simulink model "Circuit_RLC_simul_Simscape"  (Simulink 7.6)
settings: Solver=ode15s  StartTime=0.0  StopTime=0.14  RelTol=1e-3
InitFcn:
  | % paramètres du circuit RLC
  | R=1;
  | L=0.01;
  | C=1e-3;
  | 
  | % fonction de transfert du 2nd ordre
  | dzeta=R*sqrt(C/L)/2;
  | w0=1/sqrt(L*C);
StopFcn:
  | close all, clc
  | load  VC_circuit_RLC_Simscape.mat
  | plot(x(1,:),x(2,:))
  | hold on
  | plot(x(1,:),x(3,:))
  | axis([0 0.14 -0.2 1.7])
  | grid
  | title('Tension aux bornes de C et échelon d''entrée')
  | xlabel('Circuit RLC - Simulation de l''inductance et de la capacité')
libraries: fl_lib x26, nesl_utility x5

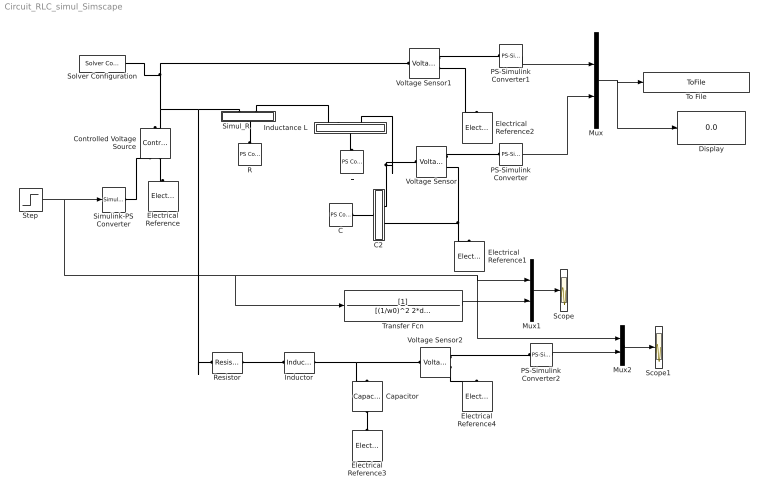
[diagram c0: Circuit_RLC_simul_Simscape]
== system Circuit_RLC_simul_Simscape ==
  C : fl_lib/Physical Signals/Sources/PS Constant  DialogController=NetworkEngine.DynNeDlgSource  SystemSampleTime=-1  constant=C  LocalVarLogging=[]
  C2 : Subsystem
  Capacitor : fl_lib/Electrical/Electrical Elements/Capacitor  DialogController=NetworkEngine.DynNeDlgSource  SystemSampleTime=-1  c=C F  v0=0 V  r=1e-6 Ohm  g=0 1/Ohm  i_Log=off  v_Log=off  vc_Log=off  LocalVarNames=|i|v|vc  LocalVarDescs=|i|v|Internal variable for voltage across capacitor term  LocalVarLogging=[0 0 0]
  Controlled Voltage Source : fl_lib/Electrical/Electrical Sources/Controlled Voltage Source  DialogController=NetworkEngine.DynNeDlgSource  SystemSampleTime=-1  i_Log=off  v_Log=off  LocalVarNames=|i|v  LocalVarDescs=|i|v  LocalVarLogging=[0 0]
  Display : Display
  Electrical Reference{,1..4} (5 alike) : fl_lib/Electrical/Electrical Elements/Electrical Reference  DialogController=NetworkEngine.DynNeDlgSource  SystemSampleTime=-1  i_Log=off  LocalVarNames=|i  LocalVarDescs=|i  LocalVarLogging=0
  "Inductance L  " : Subsystem  mask{L=0}
      mask prompts: L "Inductance"
  Inductor : fl_lib/Electrical/Electrical Elements/Inductor  DialogController=NetworkEngine.DynNeDlgSource  SystemSampleTime=-1  l=L H  i0=0 A  r=0 Ohm  g=1e-9 1/Ohm  i_Log=off  v_Log=off  i_L_Log=off  LocalVarNames=|i|v|i_L  LocalVarDescs=|i|v|Internal variable for current through inductor term  LocalVarLogging=[0 0 0]
  L : fl_lib/Physical Signals/Sources/PS Constant  DialogController=NetworkEngine.DynNeDlgSource  SystemSampleTime=-1  constant=L  LocalVarLogging=[]
  Mux : Mux  Inputs=2
  Mux1 : Mux  Inputs=2
  Mux2 : Mux  Inputs=2
  PS-Simulink Converter : nesl_utility/PS-Simulink Converter  DialogController=NetworkEngine.DynNeUtilDlgSource  SystemSampleTime=-1  PhysicalDomain=network_engine_domain  LeftPortType=input  RightPortType=output  SubClassName=ps_output  Unit=1  AffineConversion=off
  PS-Simulink Converter1 : nesl_utility/PS-Simulink Converter  DialogController=NetworkEngine.DynNeUtilDlgSource  SystemSampleTime=-1  PhysicalDomain=network_engine_domain  LeftPortType=input  RightPortType=output  SubClassName=ps_output  Unit=1  AffineConversion=off
  PS-Simulink Converter2 : nesl_utility/PS-Simulink Converter  DialogController=NetworkEngine.DynNeUtilDlgSource  SystemSampleTime=-1  PhysicalDomain=network_engine_domain  LeftPortType=input  RightPortType=output  SubClassName=ps_output  Unit=1  AffineConversion=off
  R : fl_lib/Physical Signals/Sources/PS Constant  DialogController=NetworkEngine.DynNeDlgSource  SystemSampleTime=-1  constant=R  LocalVarLogging=[]
  Resistor : fl_lib/Electrical/Electrical Elements/Resistor  DialogController=NetworkEngine.DynNeDlgSource  SystemSampleTime=-1  R=R Ohm  i_Log=off  v_Log=off  LocalVarNames=|i|v  LocalVarDescs=|i|v  LocalVarLogging=[0 0]
  Scope : Scope
  Scope1 : Scope
  Simul_R : Subsystem
  Simulink-PS Converter : nesl_utility/Simulink-PS Converter  DialogController=NetworkEngine.DynNeUtilDlgSource  SystemSampleTime=-1  PhysicalDomain=network_engine_domain  LeftPortType=input  RightPortType=output  SubClassName=ps_input  Unit=1  AffineConversion=off  InputFilterTimeConstant=.001  UdotUserProvided=0
  Solver Configuration : nesl_utility/Solver Configuration  DialogController=NetworkEngine.DynNeUtilDlgSource  SystemSampleTime=-1  PhysicalDomain=network_engine_domain  LeftPortType=input  RightPortType=generic  SubClassName=solver  Accelerate=off  Profile=off  ResidualTolerance=1e-9  MaxNonlinIter=3  MaxModeIter=2  DoFixedCost=off  UseLocalSampling=off  DoDC=off  LinearAlgebra=Sparse  LocalSolverSampleTime=.001  LocalSolverChoice=NE_BACKWARD_EULER_ADVANCER  UseLocalSolver=off
  Step : Step  Time=0.02  SampleTime=0
  To File : ToFile  Filename=VC_circuit_RLC_Simscape  MatrixName=x
  Transfer Fcn : TransferFcn  Denominator=[(1/w0)^2 2*dzeta/w0 1]
  Voltage Sensor : fl_lib/Electrical/Electrical Sensors/Voltage Sensor  DialogController=NetworkEngine.DynNeDlgSource  SystemSampleTime=-1  i1_Log=off  v1_Log=off  LocalVarNames=|i1|v1  LocalVarDescs=|i1|v1  LocalVarLogging=[0 0]
  Voltage Sensor1 : fl_lib/Electrical/Electrical Sensors/Voltage Sensor  DialogController=NetworkEngine.DynNeDlgSource  SystemSampleTime=-1  i1_Log=off  v1_Log=off  LocalVarNames=|i1|v1  LocalVarDescs=|i1|v1  LocalVarLogging=[0 0]
  Voltage Sensor2 : fl_lib/Electrical/Electrical Sensors/Voltage Sensor  DialogController=NetworkEngine.DynNeDlgSource  SystemSampleTime=-1  i1_Log=off  v1_Log=off  LocalVarNames=|i1|v1  LocalVarDescs=|i1|v1  LocalVarLogging=[0 0]
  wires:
  Mux/1 -> To File/1, Display/1
  PS-Simulink Converter/1 -> Mux/2
  PS-Simulink Converter1/1 -> Mux/1
  Step/1 -> Simulink-PS Converter/1, Transfer Fcn/1, Mux1/1, Mux2/1
  Mux1/1 -> Scope/1
  Transfer Fcn/1 -> Mux1/2
  PS-Simulink Converter2/1 -> Mux2/2
  Mux2/1 -> Scope1/1
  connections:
  Simulink-PS Converter/RConn1 -- Controlled Voltage Source/RConn1
  Controlled Voltage Source/RConn2 -- Electrical Reference/LConn1
  Simul_R/LConn1 -- Controlled Voltage Source/LConn1 -- Voltage Sensor1/LConn1 -- Solver Configuration/RConn1 -- Resistor/LConn1
  C2/RConn1 -- Voltage Sensor/LConn1 -- "Inductance L  "/RConn2
  Voltage Sensor/RConn1 -- PS-Simulink Converter/LConn1
  Voltage Sensor1/RConn1 -- PS-Simulink Converter1/LConn1
  Voltage Sensor1/RConn2 -- Electrical Reference2/LConn1
  C/RConn1 -- C2/LConn1
  "Inductance L  "/LConn1 -- L/RConn1
  C2/RConn2 -- Electrical Reference1/LConn1 -- Voltage Sensor/RConn2
  R/RConn1 -- Simul_R/RConn1
  Simul_R/LConn2 -- "Inductance L  "/RConn1
  Resistor/RConn1 -- Inductor/LConn1
  Inductor/RConn1 -- Capacitor/RConn1 -- Voltage Sensor2/LConn1
  Capacitor/LConn1 -- Electrical Reference3/LConn1
  Voltage Sensor2/RConn2 -- Electrical Reference4/LConn1
  Voltage Sensor2/RConn1 -- PS-Simulink Converter2/LConn1

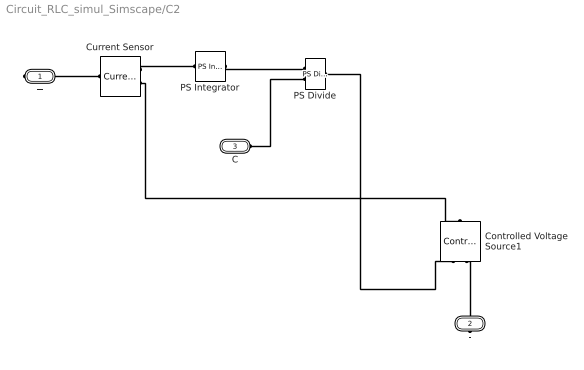
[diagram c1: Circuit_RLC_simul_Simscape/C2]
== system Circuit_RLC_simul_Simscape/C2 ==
  Controlled Voltage Source1 : fl_lib/Electrical/Electrical Sources/Controlled Voltage Source  DialogController=NetworkEngine.DynNeDlgSource  SystemSampleTime=-1  i_Log=off  v_Log=off  LocalVarNames=|i|v  LocalVarDescs=|i|v  LocalVarLogging=[0 0]
  Current Sensor : fl_lib/Electrical/Electrical Sensors/Current Sensor  DialogController=NetworkEngine.DynNeDlgSource  SystemSampleTime=-1  i1_Log=off  v1_Log=off  LocalVarNames=|i1|v1  LocalVarDescs=|i1|v1  LocalVarLogging=[0 0]
  PS Divide : fl_lib/Physical Signals/Functions/PS Divide  DialogController=NetworkEngine.DynNeDlgSource  SystemSampleTime=-1  LocalVarLogging=[]
  PS Integrator : fl_lib/Physical Signals/Linear Operators/PS Integrator  DialogController=NetworkEngine.DynNeDlgSource  SystemSampleTime=-1  x0=0  x_Log=off  LocalVarNames=|x  LocalVarDescs=|x  LocalVarLogging=0
  + : PMIOPort  Port=1  Side=Right
  - : PMIOPort  Port=2  Side=Right
  C : PMIOPort  Port=3  Side=Left
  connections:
  Current Sensor/RConn2 -- Controlled Voltage Source1/LConn1
  PS Divide/RConn1 -- Controlled Voltage Source1/RConn1
  Current Sensor/RConn1 -- PS Integrator/LConn1
  PS Integrator/RConn1 -- PS Divide/LConn1
  C/RConn1 -- PS Divide/LConn2
  +/RConn1 -- Current Sensor/LConn1
  -/RConn1 -- Controlled Voltage Source1/RConn2

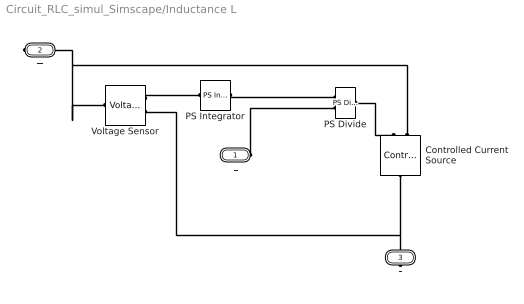
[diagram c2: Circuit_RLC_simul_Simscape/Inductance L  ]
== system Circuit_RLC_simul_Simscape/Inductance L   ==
  Controlled Current Source : fl_lib/Electrical/Electrical Sources/Controlled Current Source  DialogController=NetworkEngine.DynNeDlgSource  SystemSampleTime=-1  i_Log=off  v_Log=off  LocalVarNames=|i|v  LocalVarDescs=|i|v  LocalVarLogging=[0 0]
  PS Divide : fl_lib/Physical Signals/Functions/PS Divide  DialogController=NetworkEngine.DynNeDlgSource  SystemSampleTime=-1  LocalVarLogging=[]
  PS Integrator : fl_lib/Physical Signals/Linear Operators/PS Integrator  DialogController=NetworkEngine.DynNeDlgSource  SystemSampleTime=-1  x0=0  x_Log=off  LocalVarNames=|x  LocalVarDescs=|x  LocalVarLogging=0
  Voltage Sensor : fl_lib/Electrical/Electrical Sensors/Voltage Sensor  DialogController=NetworkEngine.DynNeDlgSource  SystemSampleTime=-1  i1_Log=off  v1_Log=off  LocalVarNames=|i1|v1  LocalVarDescs=|i1|v1  LocalVarLogging=[0 0]
  L : PMIOPort  Port=1  Side=Left
  + : PMIOPort  Port=2  Side=Right
  - : PMIOPort  Port=3  Side=Right
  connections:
  PS Divide/RConn1 -- Controlled Current Source/RConn1
  Controlled Current Source/RConn2 -- +/RConn1 -- Voltage Sensor/LConn1
  PS Integrator/RConn1 -- PS Divide/LConn1
  Voltage Sensor/RConn1 -- PS Integrator/LConn1
  L/RConn1 -- PS Divide/LConn2
  -/RConn1 -- Controlled Current Source/LConn1 -- Voltage Sensor/RConn2

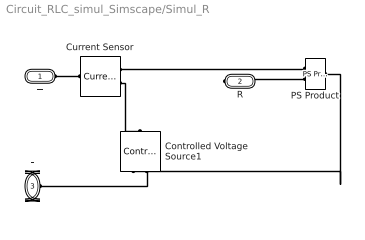
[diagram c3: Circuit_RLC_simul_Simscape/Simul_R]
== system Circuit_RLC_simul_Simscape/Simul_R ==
  Controlled Voltage Source1 : fl_lib/Electrical/Electrical Sources/Controlled Voltage Source  DialogController=NetworkEngine.DynNeDlgSource  SystemSampleTime=-1  i_Log=off  v_Log=off  LocalVarNames=|i|v  LocalVarDescs=|i|v  LocalVarLogging=[0 0]
  Current Sensor : fl_lib/Electrical/Electrical Sensors/Current Sensor  DialogController=NetworkEngine.DynNeDlgSource  SystemSampleTime=-1  i1_Log=off  v1_Log=off  LocalVarNames=|i1|v1  LocalVarDescs=|i1|v1  LocalVarLogging=[0 0]
  PS Product : fl_lib/Physical Signals/Functions/PS Product  DialogController=NetworkEngine.DynNeDlgSource  SystemSampleTime=-1  LocalVarLogging=[]
  + : PMIOPort  Port=1  Side=Left
  R : PMIOPort  Port=2  Side=Right
  - : PMIOPort  Port=3  Side=Left
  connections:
  Controlled Voltage Source1/RConn2 -- -/RConn1
  R/RConn1 -- PS Product/LConn2
  +/RConn1 -- Current Sensor/LConn1
  Current Sensor/RConn1 -- PS Product/LConn1
  PS Product/RConn1 -- Controlled Voltage Source1/RConn1
  Current Sensor/RConn2 -- Controlled Voltage Source1/LConn1
